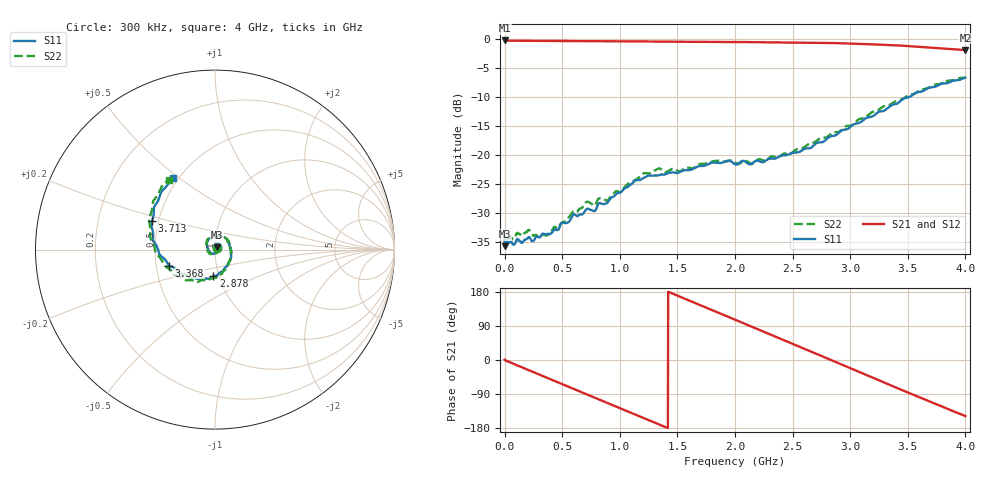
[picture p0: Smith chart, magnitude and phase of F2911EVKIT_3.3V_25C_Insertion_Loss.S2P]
! Integrated Device Technology
! Corporate Headquarters
! 6024 Silver Creek Valley Road
! San Jose, CA 95138  USA
! Phone:  1-408-284-8200
! Toll Free:  1-800-223-1366
! Webpage:  http://www.idt.com/
! Timing and RF Division
! 515 Groton Road, Suite 102
! Westford, MA 01886-6024
! Device:  F2911
! Description: 75 Ohm SPST RF Switch
! Frequency:  300 kHz to 4 GHz
! Package:  2 mm x 2 mm DFN Plastic Package: 8-pin
! Ports:  2 RF, 2 DC
!  Pin  1  = NC
!  Pin  2  = GND
!  Pin  3  = GND
!  Pin  4  = NC
!  Pin  5  = RF1	= Port 1
!  Pin  6  = VDD
!  Pin  7  = V1
!  Pin  8  = RF2	= Port 2
!  EP  = GND
! State:  Insertion Loss
! EVKIT Voltages:		VCC	= +3.3 V
!  V1	= +3.3 V (Logic HIGH)
! Data:  The device was measured on the F2911 EVKit
!  using a calibrated network analyzer.
!  The results below include the EVKit RF connector and
!  PCB loss effects. The reference plane is at
!  the SMA coaxial interface. Refer to the separate
!  measured thru line.s2p file for connector and PCB loss
!  and effects.
! Misc:
! Date Measured:  2017-8-11
! Date:  2017-9-21  SJ
! Note:
!  Integrated Device Technology supplies this data as a sample
!	of measured data. Data was taken at 25 degrees C.
!  Integrated Device Technology reserves the right to change
! 	this data at anytime.
!Freq	S11:SOLT2(ON)	S21:SOLT2(ON)	S12:SOLT2(ON)	S22:SOLT2(ON)
!PortZ  Port1:75+j0  Port2:75+j0
# Hz S dB R 75
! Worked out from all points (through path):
!   1601 points, 300 kHz to 4 GHz, reference 75 ohm
!   highest |S21| = -0.22 dB at 2.8 MHz (marker M1); lowest = -1.9 dB at 4 GHz (marker M2)
!   group delay of S21, straight-line fit = 353 ps
!   lowest |S11| = -35.7 dB at 300 kHz (marker M3), VSWR 1.03, Z = 76.6 + j1.93 ohm
!   |S11| at or under -10 dB: start of sweep to 3.509 GHz
!   |S22| runs from -35.2 to -6.6 dB; largest |S21 - S12| = 0.0024
!   S11 on the Smith chart (normalised r, x): 300 kHz: 1.02, +0.03; 2.878 GHz: 0.94, -0.29; 3.368 GHz: 0.58, -0.11; 3.713 GHz: 0.46, +0.17; 4 GHz: 0.46, +0.47
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300000  -35.72 50.4  -0.22 0.6  -0.22 0.5  -35.20 38.5
2799813  -34.60 5.0  -0.22 -0.3  -0.22 -0.4  -33.74 1.1
2.027848e8  -34.30 -42.2  -0.28 -25.9  -0.28 -25.9  -33.02 -35.4
3.002775e8  -34.17 -64.2  -0.29 -38.3  -0.29 -38.3  -34.19 -54.6
4.902632e8  -31.82 -109.2  -0.31 -62.4  -0.32 -62.4  -31.76 -105.0
6.677499e8  -30.25 -141.2  -0.33 -84.9  -0.34 -84.9  -29.15 -138.3
9.702272e8  -26.71 161.1  -0.36 -123.2  -0.37 -123.2  -26.23 168.4
1.162713e9  -24.32 135.9  -0.38 -147.6  -0.39 -147.6  -23.94 135.1
1.3352e9  -23.50 116.4  -0.41 -169.3  -0.42 -169.4  -22.32 117.3
1.645177e9  -22.29 73.4  -0.46 151.5  -0.47 151.4  -22.17 68.8
1.830163e9  -21.30 52.6  -0.48 128.0  -0.49 127.9  -20.99 45.9
2.00015e9  -21.58 33.4  -0.49 106.5  -0.49 106.4  -21.24 27.1
2.155138e9  -21.34 10.2  -0.50 86.8  -0.51 86.7  -21.48 2.3
2.312627e9  -20.60 -10.4  -0.53 66.8  -0.54 66.7  -20.26 -18.7
2.6676e9  -18.63 -63.6  -0.61 21.3  -0.62 21.3  -17.97 -65.1
2.877584e9  -16.55 -93.5  -0.67 -5.7  -0.68 -5.8  -16.04 -90.0
3.087568e9  -14.36 -122.9  -0.79 -32.9  -0.80 -33.0  -13.74 -119.1
3.33505e9  -11.75 -158.3  -1.02 -64.6  -1.04 -64.7  -11.38 -153.0
3.367547e9  -11.33 -160.9  -1.04 -68.8  -1.06 -68.9  -11.05 -158.1
3.532535e9  -9.76 176.7  -1.22 -89.9  -1.24 -90.0  -9.54 -179.2
3.712522e9  -8.28 155.8  -1.48 -112.6  -1.49 -112.7  -8.03 157.3
4e9  -6.65 120.6  -1.88 -147.9  -1.89 -148.0  -6.61 123.4
